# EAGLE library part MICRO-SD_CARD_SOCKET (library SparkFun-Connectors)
microSD Socket for Transflash Push-push type µSD socket. tDoc lines correctly indicate media card edge positions when inserting (unlocked, locked, depressed). NOTE: CD1 and CD2 are connected internally, and the default detect state of the socket is detect pin to ground. SparkFun Products: WAV Trigger CAN-Bus Shield SparkFun Level Shifing microSD Breakout
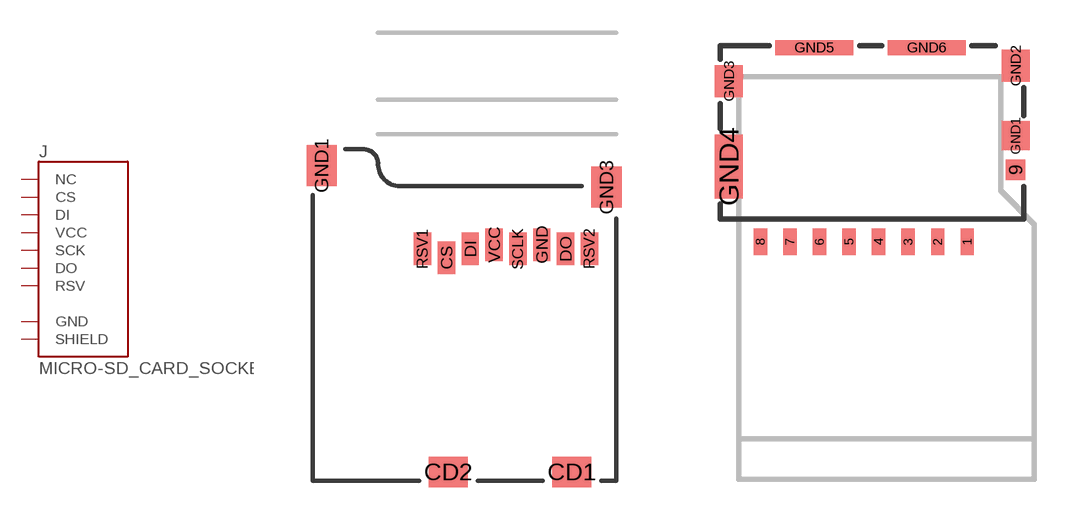
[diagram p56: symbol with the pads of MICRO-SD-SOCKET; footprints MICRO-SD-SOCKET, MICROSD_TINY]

Designator prefix J

## MICRO-SD_CARD_SOCKETPUSH-PUSH (PROD_ID: CONN-07820)  [MICRO-SD-SOCKET]
CD1  SHIELD
CS  CS
DI  DI
DO  DO
GND  GND
RSV1  RSV
RSV2  NC
SCLK  SCK
VCC  VCC

## MICRO-SD_CARD_SOCKETTINY (PROD_ID: CONN-13500)  [MICROSD_TINY]
1  RSV
2  CS
3  DI
4  VCC
5  SCK
6  GND
7  DO
8  RSV
9  NC
GND1  SHIELD
GND2  SHIELD
GND3  SHIELD
GND4  SHIELD
GND5  SHIELD
GND6  SHIELD

## Footprint MICRO-SD-SOCKET (pad centres in mm)
microSD Socket SMD Puhs-Push type. tDocu shows location of uSD card in different positions. Specifications: Pin count:12 Datasheet referenced for footprint Example device(s): MICRO-SD_CARD_SOCKET
smd 1.8 x 1.4: CD1 -2.05,0.4; CD2 -7.75,0.4
smd 0.8 x 1.5: CS -7.84,10.3; DI -6.74,10.7; DO -2.34,10.7; GND -3.44,10.9; RSV1 -8.94,10.7; RSV2 -1.24,10.7; SCLK -4.54,10.7; VCC -5.64,10.9
smd 1.4 x 1.9: GND1 -13.6,14.55; GND3 -0.45,13.55

## Footprint MICROSD_TINY (pad centres in mm)
smd 0.5 x 1: 1 9.2,-0.85; 2 8.1,-0.85; 3 7,-0.85; 4 5.9,-0.85; 5 4.8,-0.85; 6 3.7,-0.85; 7 2.6,-0.85; 8 1.5,-0.85
smd 0.72 x 0.78: 9 11,1.83
smd 1.05 x 1.08: GND1 11,3.1
smd 1.05 x 1.2: GND2 11,5.71; GND3 0.325,5.14
smd 1.05 x 2.39: GND4 0.325,1.955
smd 2.91 x 0.55: GND5 3.505,6.385; GND6 7.695,6.385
